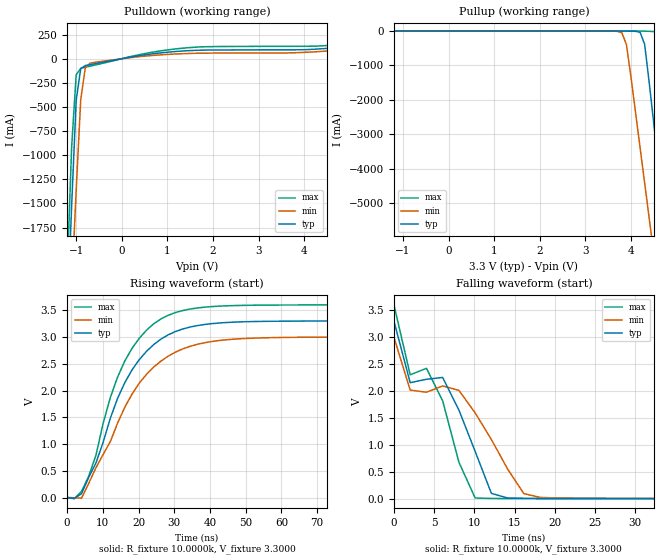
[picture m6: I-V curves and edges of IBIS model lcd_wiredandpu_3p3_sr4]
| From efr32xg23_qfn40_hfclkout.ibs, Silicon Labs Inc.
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|   Model lcd_wiredandpu_3p3_sr4
[Model]  lcd_wiredandpu_3p3_sr4
Model_type Output
Polarity   Inverting
Enable   Active-Low
C_comp   1.6300pF   1.4000pF   2.7000pF
[Temperature Range]   25.0000   0.1250k   -40.0000
[Pullup Reference]   3.3000V   3.0000V   3.6000V
[Pulldown Reference]   0.0V   0.0V   0.0V
[POWER Clamp Reference]   3.3000V   3.0000V   3.6000V
[GND Clamp Reference]   0.0V   0.0V   0.0V
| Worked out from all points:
|   slope of the pulldown table from 0 to 0.495 V, typ, clamps not added: 12.6 ohm
|   slope of the pullup table from 0 to 0.495 V, typ, clamps not added: 40.1 kohm
|   rising waveform, R_fixture 10.0000k, V_fixture 3.3000: 20-80 % time 12.9ns typ, 15.2ns min, 11.5ns max; typ from 0.004 V to 3.3 V
|   falling waveform, R_fixture 10.0000k, V_fixture 3.3000: 20-80 % time 9.5ns typ, 12.7ns min, 6.89ns max; typ from 3.3 V to 0.004 V
[Pulldown]
|Voltage   I(typ)   I(min)   I(max)
-3.3V     -27.9A     -25.09A    -30.67A
-1.2V     -2.717A    -3.413A    -2.255A
-1.1V     -1.526A    -2.386A    -916mA
-1V       -431.1mA   -1.361A    -166.1mA
-900mV    -101.3mA   -422.8mA   -99.6mA
-800mV    -71.14mA   -92.96mA   -88.1mA
-700mV    -61.69mA   -47.63mA   -77.54mA
400mV     32.64mA    21.8mA     43.42mA
1.2V      75.23mA    49.28mA    102.4mA
4.5V      107.1mA    79.44mA    136.7mA
5.5V      158.4mA    122.1mA    194.8mA
6.6V      244.6mA    192.8mA    298mA
[Pullup]
|Voltage   I(typ)   I(min)   I(max)
-3.3V     82.22uA    106.9uA    95.53uA
3.8V      -523.4uA   -50.48mA   -109.5uA
3.9V      -1.654mA   -390.8mA   -113uA
4.3V      -385.9mA   -4.417A    -4.337mA
4.4V      -1.495A    -5.447A    -8.523mA
4.5V      -2.686A    -6.476A    -15.07mA
4.6V      -3.88A     -7.507A    -84.31mA
4.7V      -5.077A    -8.538A    -881.9mA
4.8V      -6.274A    -9.569A    -2.22A
5V        -8.669A    -11.63A    -4.914A
5.1V      -9.868A    -12.66A    -6.266A
6.6V      -27.87A    -28.14A    -26.57A
[Ramp]
| variable   typ   min   max
dV/dt_r  0.3946/12.6593n   0.3211/14.1139n   0.4830/11.4424n
dV/dt_f  1.9778/9.5035n   1.7970/12.7217n   2.1582/6.8875n
R_load = 10.0000k
[Rising Waveform]
R_fixture= 10.0000k
V_fixture= 3.3000
V_fixture_min= 3.0000
V_fixture_max= 3.6000
|time   V(typ)   V(min)   V(max)
0s        3.595mV    4.859mV    2.976mV
4.04ns    73.96mV    -9.635mV   115.7mV
6.061ns   379.8mV    266.8mV    401.1mV
8.081ns   647.1mV    559mV      794mV
12.12ns   1.487V     1.05V      1.874V
18.18ns   2.386V     1.934V     2.789V
24.24ns   2.859V     2.438V     3.247V
32.32ns   3.15V      2.777V     3.494V
56.57ns   3.294V     2.988V     3.597V
200ns     3.3V       3V         3.6V
[Falling Waveform]
R_fixture= 10.0000k
V_fixture= 3.3000
V_fixture_min= 3.0000
V_fixture_max= 3.6000
|time   V(typ)   V(min)   V(max)
0s        3.3V       3V         3.6V
2.02ns    2.156V     2.019V     2.302V
4.04ns    2.22V      1.979V     2.423V
6.061ns   2.254V     2.096V     1.82V
8.081ns   1.65V      2.014V     680.9mV
10.1ns    881.9mV    1.597V     16.42mV
12.12ns   101.7mV    1.102V     7.52mV
16.16ns   9.745mV    96.87mV    5.131mV
18.18ns   7.754mV    27.21mV    4.749mV
200ns     3.596mV    4.862mV    2.977mV
